FUNCTION "AutoPress" : VOID
TITLE =Start press
VERSION : 0.1

BEGIN
NETWORK
TITLE =Ready for auto
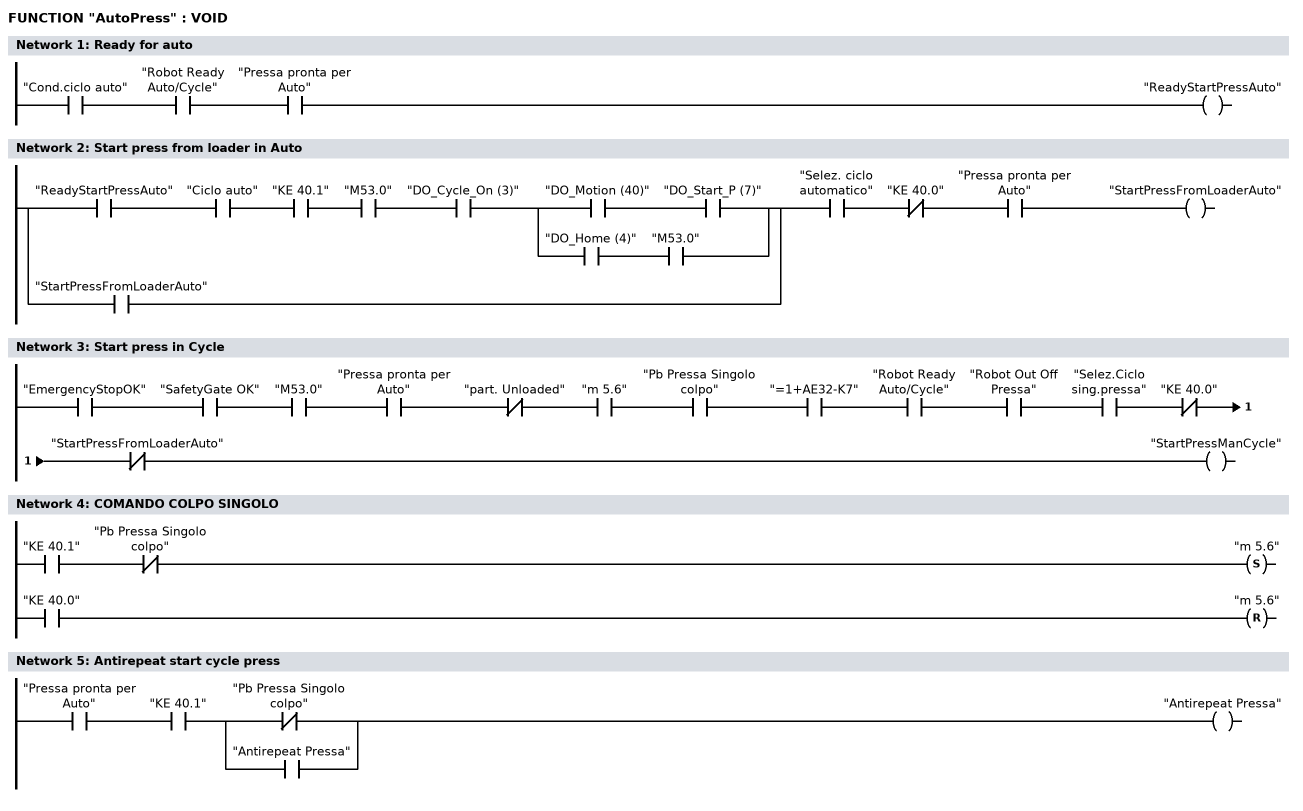
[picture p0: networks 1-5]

      U     "Cond.ciclo auto";
      U     "Robot Ready Auto/Cycle";
      U     "Pressa pronta per Auto";
      =     "ReadyStartPressAuto";
NETWORK
TITLE =Start press from loader in Auto
//
//
      U(    ;
      U     "ReadyStartPressAuto";
      U     "Ciclo auto";
      U     "KE 40.1";
      U     "M53.0";
      U     "DO_Cycle_On (3)";
      U(    ;
      U     "DO_Motion (40)";
      U     "DO_Start_P (7)";
      O     ;
      U     "DO_Home (4)";
      U     "M53.0";
      )     ;
      O     "StartPressFromLoaderAuto";
      )     ;
      U     "Selez. ciclo automatico";
      UN    "KE 40.0";
      U     "Pressa pronta per Auto";
      =     "StartPressFromLoaderAuto";
NETWORK
TITLE =Start press in Cycle
//
//
      U     "EmergencyStopOK";
      U     "SafetyGate OK";
      U     "M53.0";
      U     "Pressa pronta per Auto";
      UN    "part. Unloaded";
      U     "m 5.6";
      U     "Pb Pressa Singolo colpo";
      U     "=1+AE32-K7";
      U     "Robot Ready Auto/Cycle";
      U     "Robot Out Off Pressa";
      U     "Selez.Ciclo sing.pressa";
      UN    "KE 40.0";
      UN    "StartPressFromLoaderAuto";
      =     "StartPressManCycle";
NETWORK
TITLE =COMANDO COLPO SINGOLO

      U     "KE 40.1";
      UN    "Pb Pressa Singolo colpo";
      S     "m 5.6";
      U     "KE 40.0";
      R     "m 5.6";
      NOP   0;
NETWORK
TITLE =Antirepeat start cycle press

      U     "Pressa pronta per Auto";
      U     "KE 40.1";
      U(    ;
      ON    "Pb Pressa Singolo colpo";
      O     "Antirepeat Pressa";
      )     ;
      =     "Antirepeat Pressa";
END_FUNCTION

